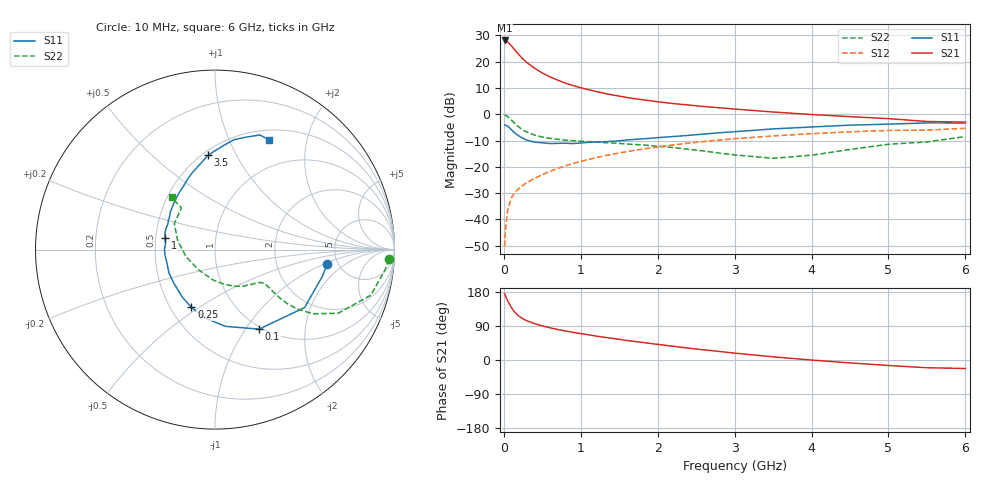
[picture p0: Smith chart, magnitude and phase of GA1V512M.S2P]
! Infineon Technologies  Discrete & RF Semiconductors
! BF775
! Si NPN RF Bipolar Junction Transistor in SOT23
! VCE = 1.5 V  IC = 12 mA
! Common Emitter S-Parameters:  May  1996
# GHz  S  MA  R  50
!  f  S11  S21  S12  S22
! GHz  MAG  ANG  MAG  ANG  MAG  ANG  MAG  ANG
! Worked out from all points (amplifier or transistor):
!   36 points, 10 MHz to 6 GHz, reference 50 ohm
!   highest |S21| = 28.1 dB at 10 MHz (marker M1)
!   |S21| within 3 dB of that: start of sweep to 124.6 MHz
!   unconditionally stable (mu >= 1): 454.8 MHz to 4.185 GHz; 5.214 GHz to end of sweep
!   at 250 MHz: K = 0.77, MSG = 24.0 dB, |S12| = -26.9 dB
!   at 1.4 GHz: K = 1.14, MAG = 9.0 dB, |S12| = -15.3 dB
!   at 6 GHz: K = 1.00, MAG = 0.8 dB, |S12| = -5.3 dB
!   S11 on the Smith chart (normalised r, x): 10 MHz: 4.10, -1.07; 100 MHz: 0.97, -1.16; 250 MHz: 0.64, -0.46; 1 GHz: 0.56, +0.08; 3.5 GHz: 0.53, +0.78; 6 GHz: 0.62, +1.42
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0.01  0.629 -7.2  25.38 175.0  0.0031 86.7  0.9707 -3.2
0.02  0.6173 -13.8  25.2 169.8  0.0061 83.9  0.9541 -6.8
0.05  0.5944 -32.9  23.79 156.2  0.0151 76.3  0.905 -16.3
0.1  0.5067 -61.0  19.87 137.8  0.0262 66.4  0.7716 -27.4
0.15  0.4308 -82.6  16.2 124.1  0.0335 61.6  0.6507 -33.3
0.2  0.3837 -98.8  13.38 115.3  0.0395 60.8  0.5644 -35.8
0.25  0.3472 -112.3  11.23 108.6  0.045 60.4  0.5024 -36.8
0.3  0.3219 -124.3  9.655 103.4  0.0502 61.2  0.4583 -36.8
0.4  0.2955 -141.3  7.518 96.0  0.0604 62.5  0.4018 -36.0
0.5  0.2872 -153.6  6.088 90.0  0.0711 63.7  0.3689 -35.1
0.6  0.2778 -164.5  5.153 84.9  0.0824 64.1  0.3488 -34.7
0.7  0.2802 -173.4  4.465 80.5  0.0933 64.5  0.3342 -34.8
0.8  0.2818 179.8  3.924 76.6  0.1044 64.3  0.3227 -35.0
1  0.2842 167.3  3.198 69.7  0.1272 63.5  0.3084 -36.6
1.1  0.2929 162.1  2.938 66.4  0.1386 63.0  0.3016 -38.1
1.3  0.2981 152.1  2.516 60.2  0.1616 61.2  0.2898 -40.7
1.6  0.3252 139.9  2.088 51.5  0.1954 58.3  0.272 -46.3
2.2  0.3772 121.4  1.601 36.2  0.2611 51.2  0.2332 -61.2
3.5  0.5273 94.2  1.106 8.4  0.3873 33.5  0.1455 -129.2
4.5  0.6214 80.2  0.901 -7.7  0.4643 19.8  0.2143 166.3
5.5  0.686 68.6  0.73 -20.4  0.5006 5.6  0.2979 129.0
6  0.6812 63.7  0.71 -22.4  0.5406 1.6  0.3769 129.6
